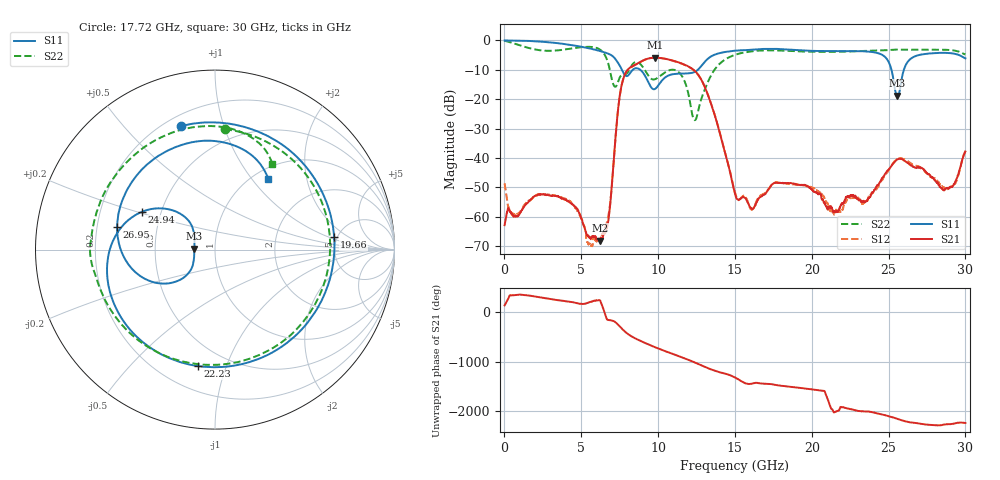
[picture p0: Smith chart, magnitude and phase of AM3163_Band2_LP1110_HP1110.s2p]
!Agilent Technologies,E8364B,MY43040894,A.07.50.67
!Agilent E8364B: A.07.50.67
!Date: Thursday, August 20, 2020 11:13:44
!Correction: S11(Full 2 Port(1,2))
!S21(Full 2 Port(1,2))
!S12(Full 2 Port(1,2))
!S22(Full 2 Port(1,2))
!S2P File: Measurements: S11, S21, S12, S22:
# Hz S  dB  R 50
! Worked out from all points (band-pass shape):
!   3201 points, 10 MHz to 30 GHz, reference 50 ohm
!   highest |S21| = -5.92 dB at 9.813 GHz (marker M1); lowest = -68.1 dB at 6.195 GHz (marker M2)
!   |S21| within 3 dB of the highest: 8.293 GHz to 11.98 GHz (3.69 GHz wide, 36.4 % of centre)
!   lowest |S11| = -18.8 dB at 25.58 GHz (marker M3), VSWR 1.26, Z = 39.7 + j0.387 ohm
!   |S11| at or under -10 dB: 7.642 GHz to 8.358 GHz (715.3 MHz wide, 8.94 % of centre); 8.835 GHz to 12.59 GHz (3.757 GHz wide, 35.1 % of centre); 25.19 GHz to 26 GHz (808.8 MHz wide, 3.16 % of centre)
!   |S22| runs from -27.2 to -0.2 dB; largest |S21 - S12| = 0.0052
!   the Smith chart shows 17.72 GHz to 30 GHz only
!   S11 on the Smith chart (normalised r, x): 17.72 GHz: 0.26, +0.73; 19.66 GHz: 4.70, +1.19; 22.23 GHz: 0.35, -0.80; 24.94 GHz: 0.39, +0.21; 26.95 GHz: 0.29, +0.10; 30 GHz: 1.17, +1.21
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1e7  -0.06 -2.5  -62.84 141.3  -48.61 -172.6  -0.18 -7.4
8.722125e8  -0.11 -31.5  -59.69 -1.6  -59.00 -4.3  -1.49 -85.1
1.903119e9  -0.31 -68.7  -53.24 -34.4  -53.32 -35.2  -3.03 -171.4
3.365131e9  -0.92 -122.4  -52.93 -108.3  -52.91 -107.8  -3.48 82.7
5.014581e9  -2.20 171.6  -60.68 173.3  -60.61 168.4  -2.35 -24.1
6.195438e9  -3.61 111.1  -68.06 -114.7  -68.38 47.3  -3.09 -111.6
7.741797e9  -11.02 -9.9  -12.97 -2.0  -13.05 -1.9  -11.58 -80.1
8.688356e9  -9.58 -75.3  -7.81 165.2  -7.87 165.6  -7.52 -129.1
9.812981e9  -16.50 -142.2  -5.92 11.9  -5.94 12.1  -13.21 -150.2
1.000979e10  -15.37 -145.6  -5.96 -12.5  -5.97 -12.3  -12.58 -149.2
1.13406e10  -11.34 91.1  -7.53 -167.4  -7.60 -167.0  -10.83 145.9
1.278387e10  -8.92 -9.1  -13.14 9.0  -13.15 10.3  -20.41 98.1
1.5005e10  -3.53 -131.2  -52.24 120.4  -51.83 119.9  -4.95 -145.1
1.772284e10  -2.93 105.4  -48.41 -35.4  -48.32 -36.5  -3.45 85.3
1.966282e10  -3.51 6.0  -49.44 -107.7  -49.61 -106.0  -3.87 -2.2
2.000958e10  -3.59 -10.4  -50.65 -119.5  -50.12 -121.7  -3.92 -16.4
2.223072e10  -3.66 -98.3  -53.42 -138.1  -54.67 -139.1  -3.83 -93.6
2.493919e10  -6.76 152.8  -44.24 60.9  -44.73 61.1  -3.36 -166.2
2.500479e10  -7.36 148.5  -43.98 55.9  -44.11 57.0  -3.34 -167.7
2.557648e10  -18.82 177.6  -40.47 0.8  -40.46 3.5  -3.17 176.9
2.695414e10  -5.04 167.1  -43.22 -91.8  -42.91 -90.5  -3.20 142.0
3e10  -6.14 52.8  -37.82 -81.0  -37.58 -82.6  -4.82 56.1
